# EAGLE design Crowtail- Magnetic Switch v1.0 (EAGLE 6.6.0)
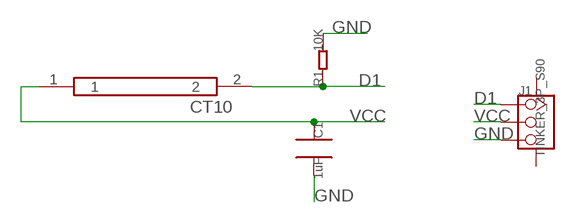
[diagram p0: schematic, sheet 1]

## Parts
C1  1uF  C0805  [0805]
J1  TINKER_3P_S90  [TINKER_3P_S90]
R1  10K  R0805  [0805]
U$1  REED-SWITCH  [REED-SWITCH]

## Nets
D1: J1.1 R1.1 U$1.2
GND: C1.2 J1.3 R1.2
VCC: C1.1 J1.2 U$1.1
Unconnected: J1.SS1 J1.SS2

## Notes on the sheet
- CT10

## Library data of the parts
C1 = CPT_SMD:C0805
J1 = Connector:TINKER_3P_S90
R1 = CPT_SMD:R0805
U$1 = seed-switch:REED-SWITCH

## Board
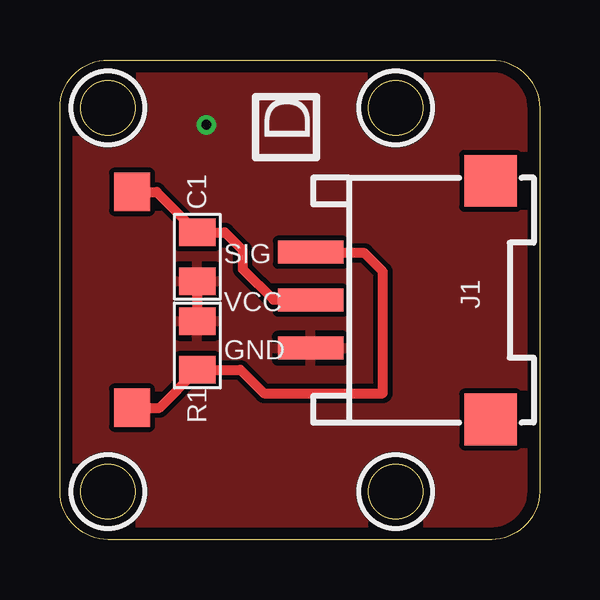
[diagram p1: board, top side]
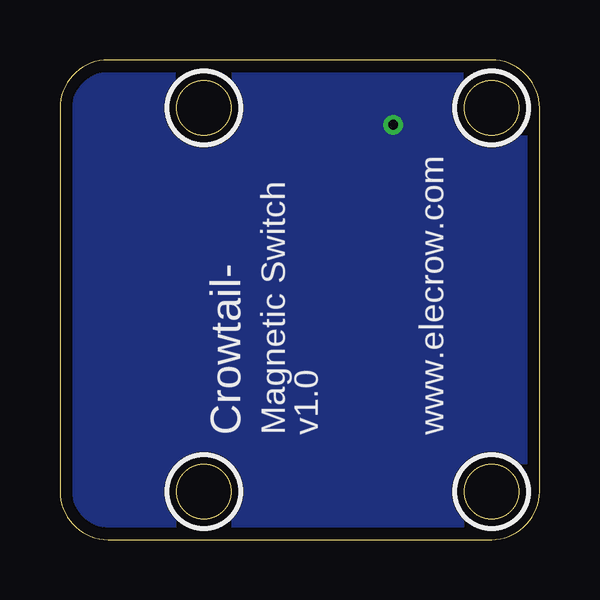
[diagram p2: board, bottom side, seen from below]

Size 20 x 20 mm. Coordinates in mm from the lower left corner, seen from the top.
Outline: 2,20 18,20 arc-90 20,18 20,2 arc-90 18,0 2,0 arc-90 0,2 0,18 arc-90 2,20
Outline: circle at 14,18 radius 1.14
Outline: circle at 14,2 radius 1.14
Outline: circle at 2,2 radius 1.14
Outline: circle at 2,18 radius 1.14
Copper layers (1*16): Top 0.035mm / dielectric 1.5mm / Bottom 0.035mm
Design rules: minimum track width 10mil, minimum drill 10mil, track to track 8mil, track to pad 8mil, pad to pad 8mil, via to via 8mil, smd to smd 8mil, copper to edge 20mil, drill to drill 10mil, minimum pad ring 10mil, minimum via ring 8mil, stop-mask expansion 4mil, vias tented up to drill 100mil, thermal gap 10mil
tRestrict: area 12.5,16.5 to 15.5,19.5; area 12.5,0.5 to 15.5,3.5; area 0.5,0.5 to 3.5,3.5; area 0.5,16.5 to 3.5,19.5
bRestrict: area 12.5,16.5 to 15.5,19.5; area 12.5,0.5 to 15.5,3.5; area 0.5,0.5 to 3.5,3.5; area 0.5,16.5 to 3.5,19.5

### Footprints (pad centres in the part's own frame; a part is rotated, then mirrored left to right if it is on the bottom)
0805 = smd 1.143 x 1.524: 1 -1.016,0; 2 1.016,0
TINKER_3P_S90 = smd 0.965 x 2.74: 1 -1.984,-4.545; 2 0.016,-4.545; 3 2.016,-4.545 | smd 2.159 x 2.184: SS1 -4.958,2.955; SS2 4.99,2.955
REED-SWITCH = smd 1.6 x 1.5: 1 -4.5,0; 2 4.5,0

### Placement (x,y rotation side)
C1  5.72,11.79 270 top
J1  15,10 270 top
R1  5.72,8.09 90 top
U$1  3,10 270 top

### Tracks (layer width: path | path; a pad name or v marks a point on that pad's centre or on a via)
D1
  Top 0.406: U$1.2 4.15,5.5 R1.1 7.53,7.08 8.51,6.1 13.46,6.1 13.46,11.18 12.7,11.94 10.5,11.94 J1.1
GND  (via drill 0.41)
  Top 0.406: C1.2 R1.2
  other vias: 6.1,17.3
  pour Top: -1.4,21.59 21.59,21.59 21.59,-1.14 -1.27,-1.14 -1.4,17.91
  pour Bottom: -1.27,-1.14 21.59,-1.27 21.59,21.59 -1.4,21.59
VCC
  Top 0.406: U$1.1 4.03,14.5 C1.1 6.88,12.81 7.62,12.06 7.62,11.28 8.9,10 10.44,10 J1.2

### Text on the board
tPlace: D | SIG | VCC | GND
bPlace: www.elecrow.com | v1.0 | Magnetic Switch | Crowtail-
